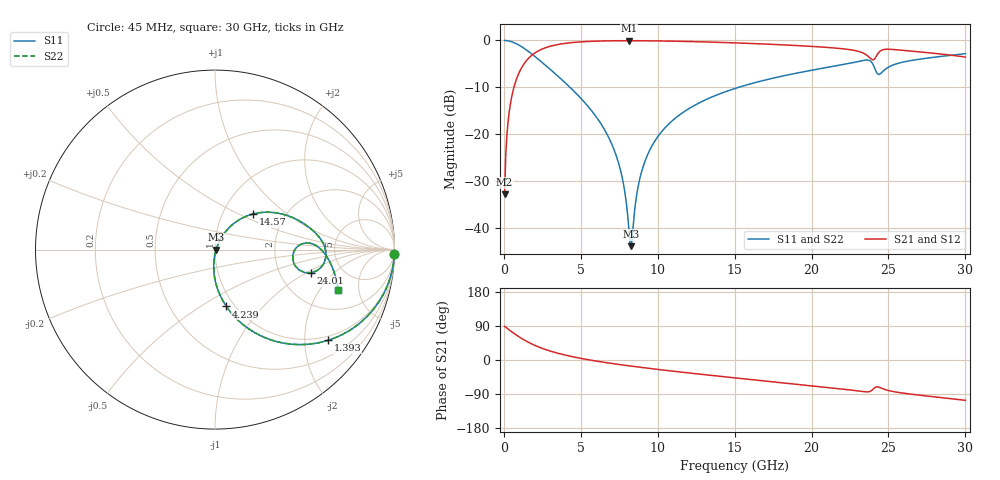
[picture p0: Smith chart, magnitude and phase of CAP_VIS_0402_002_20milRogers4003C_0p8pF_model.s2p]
! S-parameter model data by Modelithics Inc.  support@modelithics.com  813-866-6335  Tampa FL USA
! S-Parameter data specifications:
! Substrate: 20-mil Rogers 4003C, substrate thickness, H=0.508mm, Dielectric constant, Er=3.75
! PCB Mounting Pad Footprint: Pad width, PadW=0.50mm , Pad length, PadL=0.50mm , Pad gap, PadG (edge-to-edge)=0.40mm , Reference planes=1.4mm apart
! Created Wed Nov 18 12:39:15 2015
# hz S ma R 50
! 2 Port Network Data from SP1.SP block
! freq  magS11  angS11  magS21  angS21  magS12  angS12  magS22  angS22
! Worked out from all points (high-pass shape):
!   401 points, 45 MHz to 30 GHz, reference 50 ohm
!   highest |S21| = -0.06 dB at 8.133 GHz (marker M1); lowest = -32.8 dB at 45 MHz (marker M2)
!   |S21| within 3 dB of the highest: 1.852 GHz to 23.55 GHz (21.7 GHz wide, 171 % of centre); 24.26 GHz to 28.85 GHz (4.588 GHz wide, 17.3 % of centre)
!   lowest |S11| = -43.8 dB at 8.283 GHz (marker M3), VSWR 1.01, Z = 50.6 - j0.00241 ohm
!   |S11| at or under -10 dB: 4.3 GHz to 15.24 GHz (10.94 GHz wide, 112 % of centre)
!   |S22| runs from -43.8 to 0.0 dB; largest |S21 - S12| = 0
!   S11 on the Smith chart (normalised r, x): 45 MHz: 1, -82; 1.393 GHz: 0.89, -2.57; 4.239 GHz: 0.92, -0.65; 14.57 GHz: 1.39, +0.60; 24.01 GHz: 2.99, -1.11; 30 GHz: 3.18, -3.03
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4.5e7  0.9997 -1.4  0.02293 88.6  0.02293 88.6  0.9997 -1.4
2.696625e8  0.9906 -8.4  0.1363 81.6  0.1363 81.6  0.9906 -8.4
4.94325e8  0.9694 -15.1  0.2451 74.8  0.2451 74.8  0.9694 -15.1
1.392975e9  0.8069 -38.8  0.5891 51.1  0.5891 51.1  0.8069 -38.8
2.666062e9  0.5501 -61.5  0.8321 28.2  0.8321 28.2  0.5501 -61.5
4.2387e9  0.3233 -78.7  0.9421 10.6  0.9421 10.6  0.3233 -78.7
5.062462e9  0.236 -85.1  0.967 3.8  0.967 3.8  0.236 -85.1
7.2342e9  0.06375 -95.3  0.992 -10.4  0.992 -10.4  0.06375 -95.3
7.758412e9  0.0304 -92.1  0.9933 -13.4  0.9933 -13.4  0.0304 -92.1
8.13285e9  0.009347 -64.4  0.9936 -15.4  0.9936 -15.4  0.009347 -64.4
8.282625e9  0.006441 -0.2  0.9936 -16.2  0.9936 -16.2  0.006441 -0.2
8.956612e9  0.04034 61.1  0.9925 -19.7  0.9925 -19.7  0.04034 61.1
1.007992e10  0.0983 60.8  0.988 -25.2  0.988 -25.2  0.0983 60.8
1.187722e10  0.1815 54.1  0.9755 -33.6  0.9755 -33.6  0.1815 54.1
1.457318e10  0.2911 43.0  0.9478 -45.3  0.9478 -45.3  0.2911 43.0
1.50225e10  0.308 41.2  0.9423 -47.2  0.9423 -47.2  0.308 41.2
2.003996e10  0.4825 20.5  0.8637 -68.1  0.8637 -68.1  0.4825 20.5
2.28108e10  0.5863 6.5  0.7817 -80.7  0.7817 -80.7  0.5863 6.5
2.4009e10  0.5502 -13.6  0.6219 -76.8  0.6219 -76.8  0.5502 -13.6
2.438344e10  0.4344 -4.2  0.7496 -71.8  0.7496 -71.8  0.4344 -4.2
2.505742e10  0.5259 3.9  0.8056 -81.1  0.8056 -81.1  0.5259 3.9
3e10  0.7229 -18.3  0.6652 -106.4  0.6652 -106.4  0.7229 -18.3
